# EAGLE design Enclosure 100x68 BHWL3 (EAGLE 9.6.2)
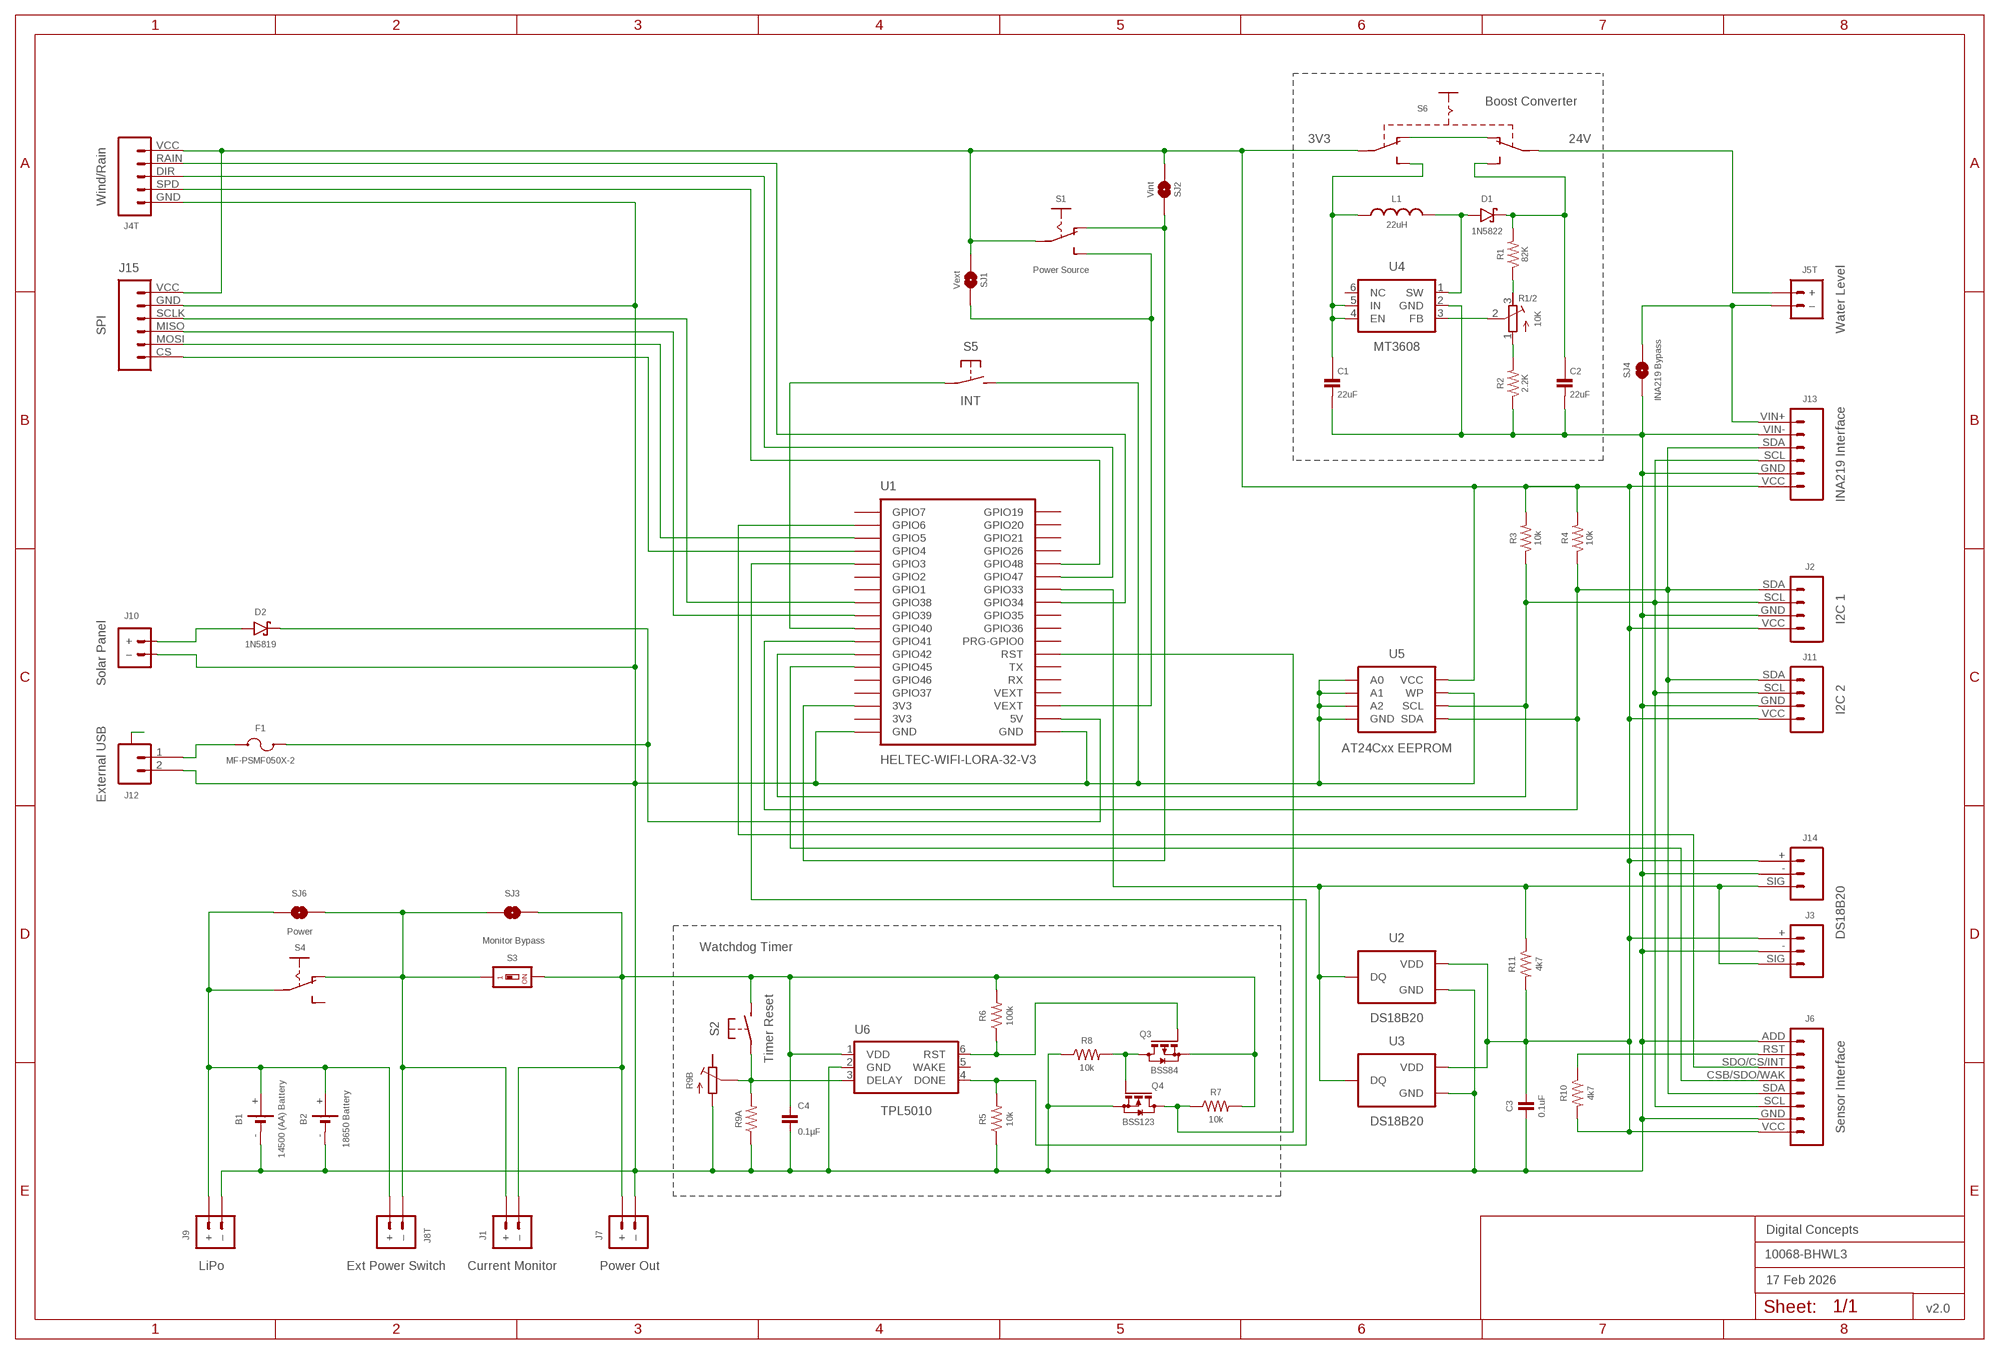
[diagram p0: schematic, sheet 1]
FRAME2 (A3L-LOC): DATE: 17 Feb 2026; OWNER: Digital Concepts; TITLE: 10068-BHWL3; VERSION: v2.0

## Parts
B1  14500 (AA) Battery  BATTERY-HOLDER-14500(AA)  [BATTERY-14500]
B2  18650 Battery  BATTERY-HOLDER-18650  [BATTERY-18650]
C1  22uF  CAPACITOR-1206  [C1206]
C2  22uF  CAPACITOR-1206  [C1206]
C3  0.1uF  CAPACITOR-0805  [C0805]
C4  0.1µF  CAPACITOR-0805  [C0805]
D1  1N5822  DIODE-SCHOTTKY-1N5822  [DIODE_SMB]
D2  1N5819  1N5819-SOD-123  [SOD-123]
F1  MF-PSMF050X-2  [F0805]
J1  Current Monitor  JST-PH2.0-2-HORIZONTALJST-PTH-2  [JST-PH2.0-2-HORIZONTAL]
J2  I2C 1  JST-PH2.0-4-VERTICAL-I2C  [JST-PH2.0-4-VERTICAL-I2C]
J3  DS18B20  JST-PH2.0-3-VERTICAL-DS18B20  [JST-PH2.0-3-VERTICAL-SIG]
J4T  Wind/Rain  JST-PH2.0-5-DUAL-WEATHER  [JST-PH2.0-5-DUAL-WEATHER]
J5T  Water Level  JST-PH2.0-2-DUAL-POWERJST-PTH-2  [JST-PH2.0-2-DUAL-POWER]
J6  Sensor Interface  HEADER-1X8-SENSOR  [CONN_08-SENSOR]
J7  Power Out  JST-GH1.25-2-HORIZONTAL-POWER  [JST-GH1.25-2-HORIZONTAL]
J8T  Ext Power Switch  JST-PH2.0-2-DUAL-POWERJST-PTH-2  [JST-PH2.0-2-DUAL-POWER]
J9  LiPo  JST-PH2.0-2-HORIZONTAL-POWERJST-PTH-2  [JST-PH2.0-2-HORIZONTAL-POWER]
J10  Solar Panel  JST-PH2.0-2-VERTICAL  [JST-PH2.0-2-VERTICAL=POWER]
J11  I2C 2  JST-PH2.0-I2C-MALE-HORIZONTAL  [JST-PH2.0-4-HORIZONTAL]
J12  External USB  JST-SH1.0-2-SMD-HORIZONTAL  [JST-SH1.0-2-HORIZONTAL]
J13  INA219 Interface  INA219-I2C-MODULE  [CONN_06-INA219]
J14  JST-PH2.0-3-HORIZONTAL-DS18B20  [JST-PH2.0-DS18B20-HORIZONTAL]
J15  SPI  JST-PH2.0-6-HORIZONTAL-SPI  [JST-PH2.0-6-HORIZONTAL-SPI]
L1  22uH  INDUCTOR-CDRH104R/6D28L5038P  [CDRH104R+6D28]
Q3  BSS84  MOSFET-BSS84  [SOT23-3]
Q4  BSS123  MOSFET-BSS123  [SOT23-3]
R1  82K  RESISTORR0805  [R0805]
R1/2  10K  RESISTOR-TRIMM-BAOTER-HORIZONTAL  [RTRIM64P]
R2  2.2K  RESISTORR0805  [R0805]
R3  10k  RESISTORR0805  [R0805]
R4  10k  RESISTORR0805  [R0805]
R5  10k  RESISTORR0805  [R0805]
R6  100k  RESISTORR0805  [R0805]
R7  10k  RESISTORR0805  [R0805]
R8  10k  RESISTORR0805  [R0805]
R9A  RESISTORR0805  [R0805]
R9B  RESISTOR-TRIMM-33  [RTRIM3*3]
R10  4k7  RESISTORR0805  [R0805]
R11  4k7  RESISTORR0805  [R0805]
S1  Power Source  SWITCH-SLIDE-SPDT-SMT  [SWITCH-SPDT-SMT]
S2  Timer Reset  SWITCH-MOMENTARY-2-PIN  [SWITCH-2-PAD]
S3  Monitor Bypass  SWITCH-DIP-SWS001  [SMD-001]
S4  Power  SWITCH-SLIDE-SPDT-PTH  [SWITCH-SPDT-PTH]
S5  INT  SWITCH-MOMENTARY-2-PIN  [SWITCH-2-PAD]
S6  SWITCH-SLIDE-DPDT-PTH-S  [SWITCH-DPDT-PTH]
SJ1  Vext  SJ  [SJ]
SJ2  Vint  SJ  [SJ]
SJ3  Monitor  SJ  [SJ]
SJ4  INA219 Bypass  SJ  [SJ]
SJ6  Power  SJ  [SJ]
U1  HELTEC-WIFI-LORA-32-V3  [HELTEC-WIFI-LORA-32-V3]
U2  DS18B20  THERMOMETER-DS18B20  [TO-92]
U3  DS18B20  THERMOMETER-DS18B20  [TO-92]
U4  MT3608  [SOT-23-6@1]
U5  AT24Cxx EEPROM  AT24CXX-EEPROM  [SOP-8]
U6  TPL5010  TPL5010DDCR  [SOT-23-6]

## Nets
A: J12.A@1(A) J12.A@2(A)
GND: B1.- B2.- C1.2 C2.2 C3.2 C4.2 J2.GND J3.- J4T.GND J6.ADD J6.GND J7.-(–) J9.-(–) J10.-(–) J11.GND J12.2 J13.GND J13.VIN- J14.- J15.GND Q4.2(S) R2.1 R5.1 R8.1 R9A.1 R9B.1(A) S5.P$2(S) SJ4.1 U1.GND@1(GND) U1.GND@36(GND) U2.1(GND) U3.1(GND) U4.2(GND) U5.P$1(A0) U5.P$2(A1) U5.P$3(A2) U5.P$4(GND) U5.P$7(WP) U6.2(GND)
N$1: D2.A J10.+
N$2: J3.SIG J14.SIG R11.1 U1.GPIO33 U2.2(DQ) U3.2(DQ)
N$3: J6.CSB/SDO/WAK U1.GPIO45
N$4: J2.SCL J6.SCL J11.SCL J13.SCL R3.1 U1.GPIO42 U5.P$6(SCL)
N$5: D2.C F1.1 U1.5V
N$6: D1.A L1.1 U4.1(SW)
N$7: Q4.3(D) R7.1 U1.RST
N$9: J6.RST R10.1
N$10: C4.1 J1.2(–) J7.+ Q3.2(S) R6.2 R7.2 S2.P$2(S) S3.2 SJ3.1 U6.1(VDD)
N$11: J2.SDA J6.SDA J11.SDA J13.SDA R4.1 U1.GPIO41 U5.P$5(SDA)
N$13: S1.3(S) SJ1.1 U1.VEXT@3(VEXT)
N$14: F1.2 J12.1
N$15: J5T.-(–) J13.VIN+ SJ4.2
N$16: S5.P$1(P) U1.GPIO40
N$17: R1.1 R1/2.3(E)
N$18: R9A.2 R9B.2(S) S2.P$1(P) U6.3(DELAY)
N$19: S1.1(O) SJ2.1 U1.3V3@34(3V3)
N$20: J5T.+ S6.P$2(P1)
N$21: J1.1(+) J8T.-(–) S3.1 S4.1(O) SJ3.2 SJ6.1
N$22: R1/2.2(S) U4.3(FB)
N$23: R1/2.1(A) R2.2
N$25: C1.1 L1.2 S6.P$6(S2) U4.4(EN) U4.5(IN)
N$26: S6.P$1(O1) S6.P$4(O2)
N$27: J15.SCLK U1.GPIO38
N$28: C2.1 D1.C R1.2 S6.P$3(S1)
N$29: J15.MOSI U1.GPIO5
N$30: B1.+ B2.+ J8T.+ J9.+ S4.2(P) SJ6.2
N$31: J15.MISO U1.GPIO39
N$32: J6.SDO/CS/INT U1.GPIO6
N$33: J15.CS U1.GPIO4
N$35: R5.2 U1.GPIO3 U6.4(DONE)
N$36: Q3.1(G) R6.1 U6.6(RST)
N$38: J4T.SPD U1.GPIO48
N$39: J4T.DIR U1.GPIO47
N$40: J4T.RAIN U1.GPIO34
N$43: Q3.3(D) Q4.1(G) R8.2
VEXT: C3.1 J2.VCC J3.+ J4T.VCC J6.VCC J11.VCC J13.VCC J14.+ J15.VCC R3.2 R4.2 R10.2 R11.2 S1.2(P) S6.P$5(P2) SJ1.2 SJ2.2 U2.3(VDD) U3.3(VDD) U5.P$8(VCC)
Unconnected: R9B.3(E) S4.3(S) U1.3V3@35(3V3) U1.GPIO0(PRG-GPIO0) U1.GPIO1 U1.GPIO2 U1.GPIO7 U1.GPIO19 U1.GPIO20 U1.GPIO21 U1.GPIO26 U1.GPIO35 U1.GPIO36 U1.GPIO37 U1.GPIO46 U1.RX U1.TX U1.VEXT@4(VEXT) U4.6(NC) U6.5(WAKE)

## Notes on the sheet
- Boost Converter
- 3V3 | 24V
- Watchdog Timer

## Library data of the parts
B1 = digitalconcepts:BATTERY-HOLDER-14500(AA): 14500 (AA) battery holder
B2 = digitalconcepts:BATTERY-HOLDER-18650: 18650 Battery Holder
C1 C2 = digitalconcepts:CAPACITOR-1206: 1206 Capacitor
C3 C4 = digitalconcepts:CAPACITOR-0805: 0805 Capacitor
D1 = digitalconcepts:DIODE-SCHOTTKY-1N5822: 1N5822 Schottky Diode SMB
D2 = digitalconcepts:1N5819-SOD-123: 1N5819 Schottky Diode SOD-123
F1 = digitalconcepts:MF-PSMF050X-2: PTC Resettable Fuse
J1 = digitalconcepts:JST-PH2.0-2-HORIZONTAL: PH2.0 2P Right Angle PCB Connector; PROD_ID: CONN-09863; SKU: PRT-09914
J2 = digitalconcepts:JST-PH2.0-4-VERTICAL-I2C: PH2.0 4P I2C Vertical Connector
J3 = digitalconcepts:JST-PH2.0-3-VERTICAL-DS18B20: DS18B20 PH2.0 Vertical PCB Connector
J4T = digitalconcepts:JST-PH2.0-5-DUAL-WEATHER: PH2.0 5P Dual Connector
J5T J8T = digitalconcepts:JST-PH2.0-2-DUAL-POWER: JST PH2.0 2P PTH Dual-Side Connector (Power); PROD_ID: CONN-09863; SKU: PRT-09914
J6 = digitalconcepts:HEADER-1X8-SENSOR: IoT Sensors 1x8 Pin Header for 'Sandwich' IoT Sensors
J7 = digitalconcepts:JST-GH1.25-2-HORIZONTAL-POWER: JST GH1.25 2P PTH Connector (Power)
J9 = digitalconcepts:JST-PH2.0-2-HORIZONTAL-POWER: PH2.0 2P Right Angle PCB Connector; PROD_ID: CONN-09863; SKU: PRT-09914
J10 = digitalconcepts:JST-PH2.0-2-VERTICAL: PH2.0 2P PCB Connector
J11 = digitalconcepts:JST-PH2.0-I2C-MALE-HORIZONTAL: PH2.0 4P (I2C) Right Angle PCB Connector
J12 = digitalconcepts:JST-SH1.0-2-SMD-HORIZONTAL: JST SH1.0 2P SMD Horizontal Connector
J13 = digitalconcepts:INA219-I2C-MODULE: INA219 I2C Module
J14 = digitalconcepts:JST-PH2.0-3-HORIZONTAL-DS18B20: DS18B20 PH2.0 Right Angle PCB Connector
J15 = digitalconcepts:JST-PH2.0-6-HORIZONTAL-SPI: PH2.0 6P Horizontal Connector—SPI
L1 = digitalconcepts:INDUCTOR-CDRH104R/6D28: Inductor; SPICEPREFIX: L
Q3 = digitalconcepts:MOSFET-BSS84: P-CHANNEL MOS FET
Q4 = digitalconcepts:MOSFET-BSS123: N-CHANNEL MOS FET
R1-R8 R9A R10 R11 = digitalconcepts:RESISTOR: Resistor; SPICEPREFIX: R
R1/2 = digitalconcepts:RESISTOR-TRIMM-BAOTER-HORIZONTAL: Trimm Resistor - Horizontal BAOTER
R9B = digitalconcepts:RESISTOR-TRIMM-3*3: Trimm Resistor - 3*3 SMD
S1 = digitalconcepts:SWITCH-SLIDE-SPDT-SMT: Mini Sliding Switch SPDT SMT
S2 S5 = digitalconcepts:SWITCH-MOMENTARY-2-PIN: 2 Pin Momentary Switch
S3 = digitalconcepts:SWITCH-DIP-SWS001: SMD Dip Switch 1 pol.
S4 = digitalconcepts:SWITCH-SLIDE-SPDT-PTH: Mini Sliding Switch SPDT PTH
S6 = digitalconcepts:SWITCH-SLIDE-DPDT-PTH-S: Switch DPDT PTH-S
SJ1-SJ4 SJ6 = digitalconcepts:SJ: Solder Jumper
U1 = digitalconcepts:HELTEC-WIFI-LORA-32-V3: Heltec WiFi LoRa 32 Development Board V3
U2 U3 = digitalconcepts:THERMOMETER-DS18B20: Digital Thermometer -55C-125C TO92-3; AVAILABILITY: Bad; DESCRIPTION: Temperature Sensor Digital, Local -55°C ~ 125°C 12 b 8-uMAX; MF: Maxim Integrated; MP: DS18B20; PACKAGE: TO-92 Maxim Integrated; PRICE: None
U4 = digitalconcepts:MT3608: MT3608 DC-DC Step-Up Voltage Converter
U5 = digitalconcepts:AT24CXX-EEPROM: AT24Cxx EEPROM SOP-8
U6 = digitalconcepts:TPL5010DDCR: TPL5010 Nano-Power System Timer with Watchdog

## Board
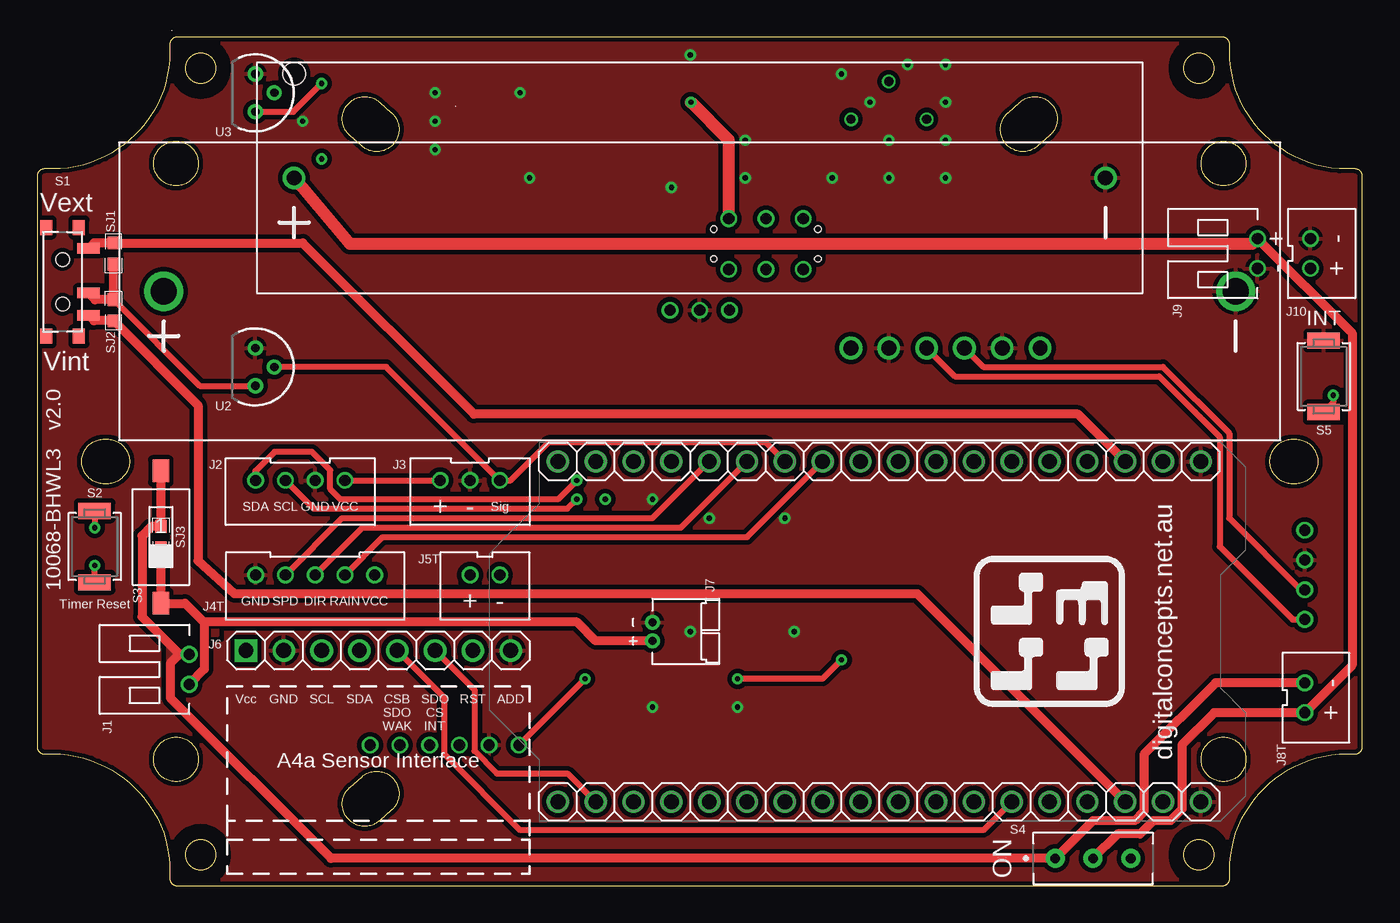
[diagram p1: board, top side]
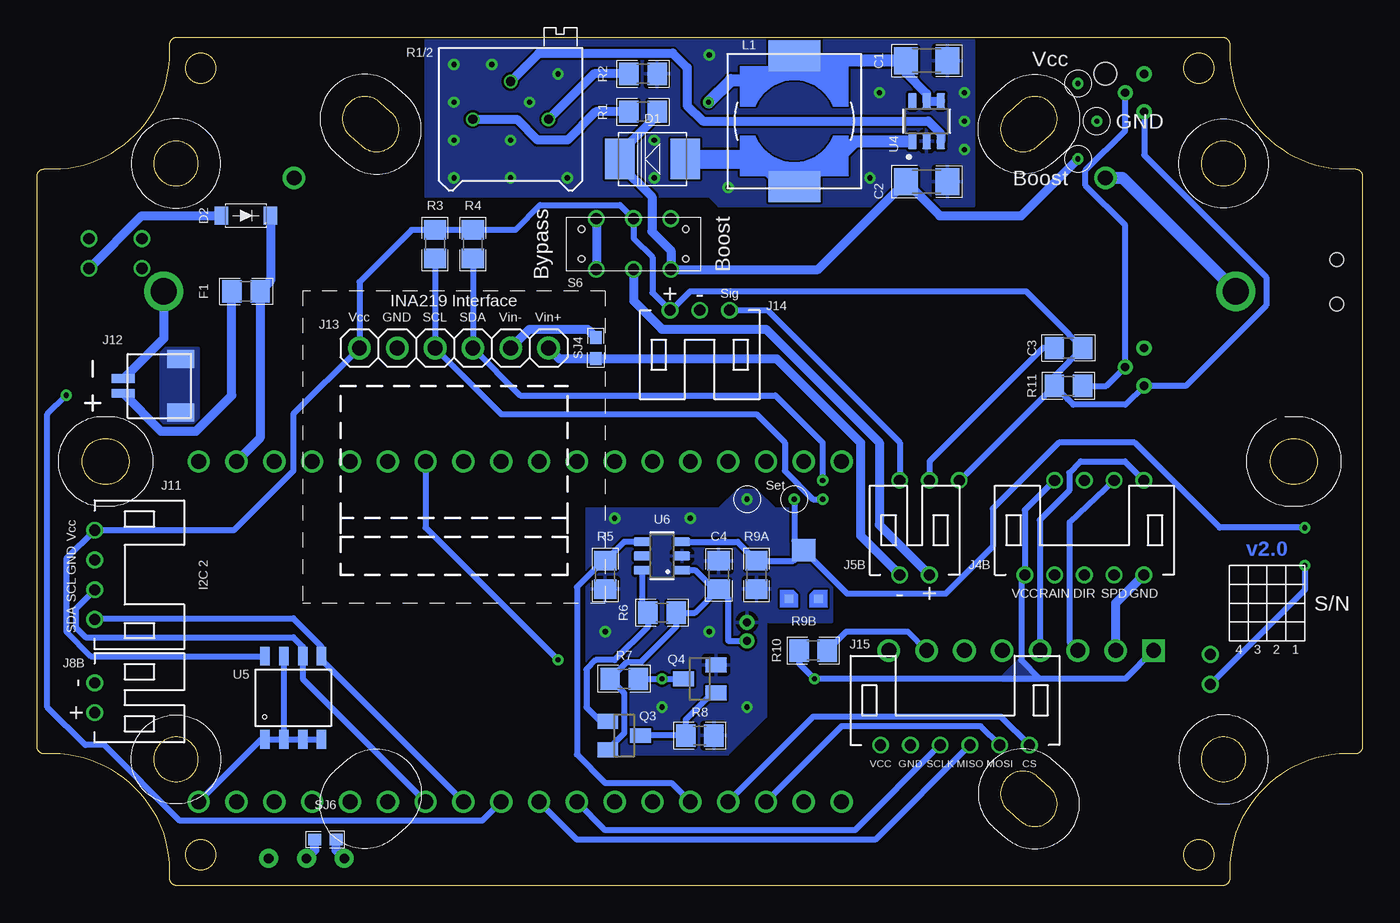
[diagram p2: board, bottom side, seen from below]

Size 89 x 57 mm. Coordinates in mm from the lower left corner, seen from the top.
Outline: 1134 segments
Outline: circle at 10.97,2.08 radius 1.02
Outline: circle at 10.97,54.92 radius 1.02
Outline: circle at 78.03,54.92 radius 1.02
Outline: circle at 78.03,2.08 radius 1.02
Copper layers (1*16): Top 0.035mm / dielectric 1.5mm / Bottom 0.035mm
Design rules "default *": minimum track width 6mil, minimum drill 0.35mm, track to track 6mil, track to pad 6mil, pad to pad 6mil, via to via 6mil, smd to smd 6mil, copper to edge 6mil, drill to drill 6mil, minimum pad ring 1mil, minimum via ring 8mil, stop-mask expansion 4mil, vias tented up to drill 0mil, thermal gap 10mil

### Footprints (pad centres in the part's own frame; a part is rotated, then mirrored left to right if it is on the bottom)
BATTERY-14500 = drill 1: + -27.25,0; - 27.25,0 | hole 1.524: -27.25,7
BATTERY-18650 = drill 1.75: + -36,0; - 36,0
C1206 = smd 1.6 x 1.8: 1 -1.4,0; 2 1.4,0
C0805 = smd 1.3 x 1.5: 1 -0.95,0; 2 0.95,0
DIODE_SMB = smd 2 x 2.7: A 2.2,0; C -2.2,0
SOD-123 = smd 0.91 x 1.22: A -1.65,0; C 1.65,0
F0805 = smd 1.3 x 1.5: 1 -0.95,0; 2 0.95,0
JST-PH2.0-2-HORIZONTAL = drill 0.75: 1 1,0; 2 -1,0
JST-PH2.0-4-VERTICAL-I2C = drill 0.75: GND 1,0; SCL -1,0; SDA -3,0; VCC 3,0
JST-PH2.0-3-VERTICAL-SIG = drill 0.75: + -2,0; - 0,0; SIG 2,0
JST-PH2.0-5-DUAL-WEATHER = drill 0.75: DIR 0,0; GND 4,0; RAIN -2,0; SPD 2,0; VCC -4,0
JST-PH2.0-2-DUAL-POWER = drill 0.75: + 1,0; - -1,0
CONN_08-SENSOR = drill 1 pad 1.524: ADD 17.78,0; CSB/SDO/WAK 10.16,0; GND 2.54,0; RST 15.24,0; SCL 5.08,0; SDA 7.62,0; SDO/CS/INT 12.7,0 | drill 1 pad 1.524 square: VCC 0,0
JST-GH1.25-2-HORIZONTAL = drill 0.55 pad 1.016: + -0.625,0; - 0.625,0
JST-PH2.0-2-HORIZONTAL-POWER = drill 0.75: + 1,0; - -1,0
JST-PH2.0-2-VERTICAL=POWER = drill 0.75: + -1,0; - 1,0
JST-PH2.0-4-HORIZONTAL = drill 0.75: GND -1,0; SCL 1,0; SDA 3,0; VCC -3,0
JST-SH1.0-2-HORIZONTAL = smd 0.6 x 1.55: 1 -0.5,2.54; 2 0.5,2.54 | smd 1.2 x 1.8: A@1 -1.8,-1.335; A@2 1.8,-1.335
CONN_06-INA219 = drill 1 pad 1.524: GND 2.54,0; SCL 5.08,0; SDA 7.62,0; VCC 0,0; VIN+ 12.7,0; VIN- 10.16,0
JST-PH2.0-DS18B20-HORIZONTAL = drill 0.75: + 2,0; - 0,0; SIG -2,0
JST-PH2.0-6-HORIZONTAL-SPI = drill 0.75: CS 5,0; GND -3,0; MISO 1,0; MOSI 3,0; SCLK -1,0; VCC -5,0
CDRH104R+6D28 = smd 2.1 x 3.5: 1 -4.4,0; 2 4.4,0
SOT23-3 = smd 1 x 1.4: 1 -0.95,-1.1; 2 0.95,-1.1; 3 0,1.1
R0805 = smd 1.3 x 1.5: 1 -0.95,0; 2 0.95,0
RTRIM64P = drill 0.61: 1 0,-2.54; 2 2.54,0; 3 0,2.54
RTRIM3*3 = smd 0.6 x 0.6: 1 -1,-1.6; 3 1,-1.6 | smd 1.6 x 1.5: 2 0,1.65
SWITCH-SPDT-SMT = smd 0.7 x 1.5: 1 2.25,1.75; 2 0.75,1.75; 3 -2.25,1.75 | smd 1 x 0.8: GND@1 3.65,-1.1; GND@2 3.65,1.1; GND@3 -3.65,1.1; GND@4 -3.65,-1.1 | hole 0.9: -1.5,0; 1.5,0
SWITCH-2-PAD = smd 1.067 x 2.184: P$1 -2.4,0; P$2 2.4,0
SMD-001 = smd 1.1 x 1.5: 1 0,-4.45; 2 0,4.45
SWITCH-SPDT-PTH = drill 0.65 pad 1.27: 1 -2.54,0; 2 0,0; 3 2.54,0
SWITCH-DPDT-PTH = drill 0.75: P$1 -1.7,2.5; P$2 -1.7,0; P$3 -1.7,-2.5; P$4 1.7,2.5; P$5 1.7,0; P$6 1.7,-2.5 | hole 0.42: 1,3.5; -1,3.5; 1,-3.5; -1,-3.5
SJ = smd 0.864 x 0.762: 1 -0.711,0; 2 0.711,0
HELTEC-WIFI-LORA-32-V3 = drill 1: 3V3@34 -22.86,5.08; 3V3@35 -22.86,2.54; 5V 0,2.54; GND@1 0,0; GND@36 -22.86,0; GPIO0 0,17.78; GPIO1 -22.86,27.94; GPIO2 -22.86,30.48; GPIO3 -22.86,33.02; GPIO4 -22.86,35.56; GPIO5 -22.86,38.1; GPIO6 -22.86,40.64; GPIO7 -22.86,43.18; GPIO19 0,43.18; GPIO20 0,40.64; GPIO21 0,38.1; GPIO26 0,35.56; GPIO33 0,27.94; GPIO34 0,25.4; GPIO35 0,22.86; GPIO36 0,20.32; GPIO37 -22.86,7.62; GPIO38 -22.86,25.4; GPIO39 -22.86,22.86; GPIO40 -22.86,20.32; GPIO41 -22.86,17.78; GPIO42 -22.86,15.24; GPIO45 -22.86,12.7; GPIO46 -22.86,10.16; GPIO47 0,30.48; GPIO48 0,33.02; RST 0,15.24; RX 0,10.16; TX 0,12.7; VEXT@3 0,5.08; VEXT@4 0,7.62
TO-92 = drill 0.55 pad 1.016: 1 -1.27,0; 2 0,1.27; 3 1.27,0
SOT-23-6@1 = smd 1.1 x 0.6: 1 -1.35,0.95; 2 -1.35,0; 3 -1.35,-0.95; 4 1.35,-0.95; 5 1.35,0; 6 1.35,0.95
SOP-8 = smd 0.635 x 1.27: P$1 -1.905,-2.794; P$2 -0.635,-2.794; P$3 0.635,-2.794; P$4 1.905,-2.794; P$5 1.905,2.794; P$6 0.635,2.794; P$7 -0.635,2.794; P$8 -1.905,2.794
SOT-23-6 = smd 1.1 x 0.6: 1 -1.35,0.95; 2 -1.35,0; 3 -1.35,-0.95; 4 1.35,-0.95; 5 1.35,0; 6 1.35,0.95

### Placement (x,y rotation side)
B1  44.5,47.55 0 top
B2  44.5,39.93 0 top
C1  29.26,55.42 0 bottom
C2  29.26,47.3 0 bottom
C3  19.73,36.12 180 bottom
C4  43.23,20.88 90 bottom
D1  47.67,48.82 0 bottom
D2  74.98,45.01 0 bottom
F1  74.98,39.93 180 bottom
J1  10.21,14.53 90 top
J2  17.67,27.23 0 top
J3  29.07,27.23 0 top
J4T  18.67,20.88 0 bottom
J5T  30.07,20.88 0 bottom
J6  14.02,15.8 0 top
J7  41.32,17.07 90 top
J8T  85.14,12.62 270 bottom
J9  81.96,42.47 90 top
J10  85.52,42.47 90 top
J11  85.14,20.88 270 bottom
J12  80.69,33.58 90 bottom
J13  67.36,36.12 0 bottom
J14  44.5,38.66 180 bottom
J15  27.35,9.45 0 bottom
L1  38.15,51.36 90 bottom
Q3  49.58,10.08 270 bottom
Q4  44.5,13.89 90 bottom
R1  48.31,51.99 0 bottom
R1/2  57.2,51.49 90 bottom
R2  48.31,54.53 180 bottom
R3  62.28,43.1 90 bottom
R4  59.74,43.1 90 bottom
R5  50.85,20.88 90 bottom
R6  47.04,18.34 0 bottom
R7  49.58,13.89 180 bottom
R8  44.5,10.08 180 bottom
R9A  40.69,20.88 90 bottom
R9B  37.51,20.88 0 bottom
R10  36.88,15.8 180 bottom
R11  19.73,33.58 180 bottom
S1  1.7,40.56 270 top
S2  3.86,22.78 270 top
S3  8.3,23.42 180 top
S4  70.92,1.83 0 top
S5  86.41,34.21 90 top
S6  48.94,43.1 90 bottom
SJ1  5.13,42.47 270 top
SJ2  5.13,38.66 90 top
SJ3  8.3,23.42 90 top
SJ4  51.48,36.12 270 bottom
SJ6  69.65,3.1 180 bottom
U1  78.15,28.5 90 top
U2  14.65,34.85 270 top
U3  14.65,53.26 270 top
U4  29.26,51.36 90 bottom
U5  71.8,12.62 0 bottom
U6  47.04,22.15 180 bottom

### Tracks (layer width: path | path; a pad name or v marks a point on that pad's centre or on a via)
$X
  cutout Bottom: 10.97,56.95 arc180 10.97,52.88 arc180
$X1
  cutout Bottom: 78.03,56.95 arc180 78.03,52.88 arc180
$X2
  cutout Top: 78.03,4.12 arc180 78.03,0.05 arc180
$X3
  cutout Top: 10.97,4.12 arc180 10.97,0.05 arc180
$X4
  cutout Top: 10.97,56.95 arc180 10.97,52.88 arc180
$X5
  cutout Top: 78.03,56.95 arc180 78.03,52.88 arc180
$X6
  cutout Bottom: 78.03,4.12 arc180 78.03,0.05 arc180
$X7
  cutout Bottom: 10.97,4.12 arc180 10.97,0.05 arc180
A
  pour Bottom (no thermals): 78.15,36.12 80.69,36.12 80.69,31.04 78.15,31.04
GND  (via drill 0.35)
  Bottom 0.406: U5.P$7 U5.P$2 | U5.P$2 U5.P$1 73.96,9.83 U1.GND@36 | U5.P$2 U5.P$3 U5.P$4 | C3.2 21.45,36.12 29.07,28.5 J3.-
  Bottom 0.61: J4T.GND 16.57,18.97 16.57,15.81 J6.GND | J13.VIN- 55.93,37.39 52.04,37.39 SJ4.1 | J12.2 83.18,34.08 80.5,36.76 B2.-
  other vias: 26.72,53.26 54.02,54.53 55.93,52.63 47.55,50.09 47.55,47.55 53.39,47.55 57.2,47.55 57.2,50.09 61.01,47.55 61.01,50.09 61.01,55.17 26.72,51.36 58.47,55.17 61.01,52.63 43.86,55.8 32.43,53.26 33.07,47.55 26.72,49.45 17.83,51.36 42.59,46.91 43.86,17.07 50.85,17.07 41.32,25.96 50.21,24.69 45.13,24.69 41.32,11.99 47.04,11.99
  pour Top (isolate 0.305, rank 2): -1.65,58.87 -1.65,-1.92 90.59,-1.92 90.59,58.87
  pour Bottom: 26.08,57.07 26.08,45.64 43.23,45.64 43.86,46.28 62.91,46.28 62.91,57.07
  pour Bottom: 52.12,25.32 52.12,8.81 42.59,8.81 40.05,11.35 40.05,17.7 35.61,17.7 35.61,25.32 39.42,25.32 40.69,26.59 41.96,26.59 43.23,25.32
N$1
  Bottom 0.61: J10.+ 81.98,45.01 D2.A
N$2
  Top 0.406: U2.2 23.45,34.85 J3.SIG 31.8,27.23 34.34,29.77 48.94,29.77 U1.GPIO33
  Bottom 0.406: J3.SIG 31.07,29.77 39.96,38.66 J14.SIG | U3.2 15.92,50.72 18.59,48.06 18.59,47.04 15.92,44.37 U2.2 17.19,33.58 R11.1
N$3
  Top 0.406: J6.CSB/SDO/WAK 27.35,12.62 27.35,8.81 32.43,3.73 63.55,3.73 U1.GPIO45
N$4  (via drill 0.35)
  Top 0.406: J13.SCL 63.55,34.85 75.61,34.85 80.06,30.4 80.06,24.69 84.87,19.88 J11.SCL | J2.SCL 18.57,25.32 35.61,25.32 v36.24,25.96
  Bottom 0.406: J2.SCL 19.66,24.41 19.66,16.36 J6.SCL | J11.SCL 86.41,18.61 86.41,17.34 85.76,16.69 71.8,16.69 71.17,16.05 U5.P$6 71.17,13.89 U1.GPIO42 | R3.1 J13.SCL 57.83,31.67 40.69,31.67 38.78,29.77 38.78,27.86 36.88,25.96 v36.24,25.96
N$5
  Bottom 0.61: D2.C 73.33,40.63 F1.1 74.03,30.08 U1.5V
N$6
  Bottom 0.152: U4.1 30.4,50.01
  Bottom 0.813: 40.68,48.82 38.96,47.11 L1.1 36.84,48.27 35.79,48.27 34.05,50.01 30.4,50.01
  Bottom 1.27: D1.A 40.68,48.82
N$7  (via drill 0.35)
  Top 0.406: v54.02,15.16 52.75,13.89 v47.04,13.89
  Bottom 0.406: R7.1 v47.04,13.89 Q4.3 | U1.RST 62.91,24.05 v54.02,15.16
N$8
  pour Top: 11.48,17.7 12.75,17.7 11.48,16.43
N$9
  Bottom 0.406: R10.1 34.66,17.07 30.53,17.07 J6.RST
N$10  (via drill 0.35)
  Top 0.406: S2.P$2 v3.86,21.51
  Top 0.61: J1.2 11.23,14.55 11.23,17.67 11.19,17.7 | J7.+ 37.51,16.44 36.25,17.7 11.19,17.7 | SJ3.1 S3.2 9.93,18.97 11.19,17.7
  Bottom 0.406: C4.1 44.82,18.34 R6.2 46.09,17.38 48.47,15 49.43,15 49.64,14.79 R7.2 49.58,12.94 49.58,10.23 Q3.2 | U6.1 44.82,21.2 43.55,19.93 C4.1 | C4.1 42.59,19.29 42.59,16.44 J7.+ | J1.2 3.86,19.88 v3.86,21.51
N$11  (via drill 0.35)
  Top 0.406: J13.SDA 61.64,34.21 75.36,34.21 79.42,30.15 79.42,22.78 84.33,17.88 J11.SDA | J2.SDA 14.67,27.86 15.94,29.13 18.46,29.13 19.68,27.92 19.68,26.65 20.37,25.96 34.97,25.96 v36.24,27.23
  Bottom 0.406: J6.SDA 21.66,15.82 21.66,24.56 19.68,26.54 19.68,27.73 18.92,28.5 15.94,28.5 J2.SDA | J11.SDA 85.06,17.96 71.8,17.96 69.9,16.05 U5.P$5 69.9,15.16 U1.GPIO41 | R4.1 J13.SDA 56.56,32.94 39.42,32.94 36.24,29.77 v36.24,27.23
N$13
  Top 0.61: S1.3 3.82,43.18 SJ1.1 17.83,43.18 29.34,31.67 69.9,31.67 U1.VEXT@3
N$14
  Bottom 0.61: J12.1 80.69,30.54 78.33,30.54 75.93,32.94 F1.2
N$15
  Bottom 0.61: J5T.- 33.7,23.51 33.7,29.77 39.34,35.41 SJ4.2 53.95,35.41 J13.VIN+
N$16  (via drill 0.35)
  Top 0.406: S5.P$1 87.04,32.45 v87.04,32.94
  Bottom 0.406: v87.04,32.94 88.31,31.67 88.31,11.99 85.77,9.45 84.5,9.45 79.42,4.37 59.1,4.37 U1.GPIO40
N$17
  Bottom 0.61: R1.1 51.48,51.99 53.39,50.09 55.38,50.09 56.78,51.49 R1/2.3
N$18  (via drill 0.35)
  Top 0.406: S2.P$1 v3.86,24.05
  Bottom 0.406: U6.3 41.96,23.1 R9A.2 38.21,21.83 R9B.2 | R9B.2 34.59,19.61 27.99,19.61 24.81,22.78 24.81,25.32 20.37,29.77 15.29,29.77 9.57,24.05 v3.86,24.05 | v38.15,25.96 38.15,23.16 R9B.2
N$19
  Top 0.61: S1.1 3.82,37.95 SJ2.1 10.81,32.27 10.81,21.82 13.24,19.61 59.1,19.61 U1.3V3@34
N$20
  Bottom 0.61: S6.P$2 48.94,39.29 47.04,37.39 40.05,37.39 32.43,29.77 32.43,24.24 J5T.+
N$21
  Top 0.61: S3.1 SJ3.2 7.67,24.13 7.03,23.5 7.03,18.07 9.57,15.53 J1.1 9.55,15.53 8.94,14.92 8.94,12.62 19.73,1.83 S4.1 70.92,4.37 73.71,4.37 74.34,5 74.34,8.81 79.15,13.62 J8T.-
  Bottom 0.61: S4.1 68.93,2.39 SJ6.1
  pour Top (no thermals): 9.55,15.55 8.94,16.16 8.94,14.94
N$22
  Bottom 0.61: U4.3 28.31,50.51 29.16,51.36 44.3,51.36 45.35,52.41 45.35,54.95 46.33,55.93 55.29,55.93 R1/2.2
N$23
  Bottom 0.61: R2.2 51.61,54.53 R1/2.1
N$25  (via drill 0.35)
  Top 0.813: v43.9,52.63 46.44,50.09 S6.P$6
  Bottom 0.61: C1.1 30.66,54.61 29.26,53.21 U4.5 U4.4
  Bottom 0.813: C1.1 38.04,55.42 L1.2 38.99,55.36 39.98,54.12 42.41,54.12 v43.9,52.63
N$26
  Bottom 0.61: S6.P$4 S6.P$1
N$27
  Bottom 0.406: J15.SCLK 34.07,3.73 50.85,3.73 U1.GPIO38
N$28  (via drill 0.35)
  Bottom 0.61: v19.1,48.82 22.91,45.01 28.37,45.01 C2.1 36.55,41.4 S6.P$3 46.44,42.67 47.71,43.94 47.71,46.28 49.87,48.44 D1.C 49.87,49.23 47.36,51.74 R1.2
N$29
  Bottom 0.406: J15.MOSI 25.62,10.72 34.97,10.72 U1.GPIO5
N$30
  Top 0.61: J9.+ 88.31,37.12 88.31,14.8 J8T.+ 79.06,11.62 76.88,9.45 76.88,5.13 76.12,4.37 74.98,4.37 74.09,3.48 72.57,3.48 S4.2
  Top 0.813: J9.+ 81.6,43.1 21,43.1 B1.+
  Bottom 0.61: S4.2 70.36,2.39 SJ6.2
  Bottom 0.813: B1.+ 16.12,47.55 B2.+
N$31
  Bottom 0.406: J15.MISO 32.7,3.1 52.75,3.1 U1.GPIO39
N$32
  Top 0.406: J6.SDO/CS/INT 29.36,13.16 29.36,9.04 30.86,7.54 35.61,7.54 U1.GPIO6
N$33
  Bottom 0.406: J15.CS 24.26,11.35 36.88,11.35 U1.GPIO4
N$35
  Bottom 0.406: U1.GPIO3 46.4,6.91 50.85,6.91 52.75,8.81 52.75,20.05 50.98,21.83 R5.2 49.58,23.1 U6.4
N$36
  Bottom 0.406: U6.6 48.39,18.74 R6.1 47.99,17.39 50.21,15.16 51.48,15.16 52.12,14.53 52.12,11.99 51.16,11.03 Q3.1
N$38
  Top 0.406: J4T.SPD 20.48,24.69 41.32,24.69 U1.GPIO48
N$39
  Top 0.406: J4T.DIR 21.84,24.05 43.23,24.05 U1.GPIO47
N$40
  Top 0.406: J4T.RAIN 23.21,23.42 47.67,23.42 U1.GPIO34
N$43
  Bottom 0.406: Q3.3 R8.2 45.45,11.15 43.65,12.94 Q4.1
VEXT  (via drill 0.35)
  Top 0.406: SJ2.2 10.92,33.58 U2.3 | v19.1,53.9 17.19,51.99 U3.3 | J15.VCC v36.8,13.89 | J2.VCC J3.+
  Top 0.61: S1.2 3.89,39.37 SJ2.2 SJ1.2
  Bottom 0.406: U3.3 14.65,49.08 6.45,40.87 6.45,38.98 11.86,33.58 U2.3 15.92,32.31 19.42,32.31 19.79,32.68 19.79,32.69 R11.2 | R11.2 20.68,34.22 19.68,35.22 19.68,35.23 C3.1 19.68,37.01 19.68,37.02 22.59,39.93 45.13,39.93 46.4,38.66 J14.+ 47.67,39.83 47.67,42.22 48.94,43.49 S6.P$5 49.86,45.72 55.22,45.72 56.88,44.05 R4.2 R3.2 63.87,44.05 67.36,40.56 J13.VCC 71.8,31.67 71.8,27.86 75.79,23.88 J11.VCC 87.04,21.97 87.04,17.07 85.39,15.42 U5.P$8 | J2.VCC 22.67,25.23 J4T.VCC 22.91,20.64 22.91,15.16 21.64,13.89 | R11.2 27.03,27.23 J3.+ | R10.2 37.83,14.92 v36.8,13.89 21.64,13.89 | J6.VCC 15.92,13.89 21.64,13.89
  pour Bottom (no thermals): 22.91,15.16 24.18,13.89 21.64,13.89

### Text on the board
Bottom: v2.0
tPlace: 10068-BHWL3 v2.0 | digitalconcepts.net.au | Vcc | GND | SCL | SDA | RST | ADD | CSB / SDO / WAK | SDO / CS / INT
bPlace: Vin+ | Vin- | SDA | SCL | GND | Vcc | Set | S/N | 1 | 2 | 3 | 4
tNames: Vext | Vint | A4a Sensor Interface | ON
bNames: Vcc | GND | Boost | Boost | Bypass | Vcc | GND | J4B | J5B | SCL | SDA | J8B
tValues: Boost Out
bValues: Wind/Rain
